FUNCTION_BLOCK "Function_Call1"
VERSION : 0.1
   VAR_INPUT
      In1 : Bool;
   END_VAR


BEGIN
NETWORK
TITLE =
      CALL "__Function"
      (  param                   := #In1
      );

END_FUNCTION_BLOCK

